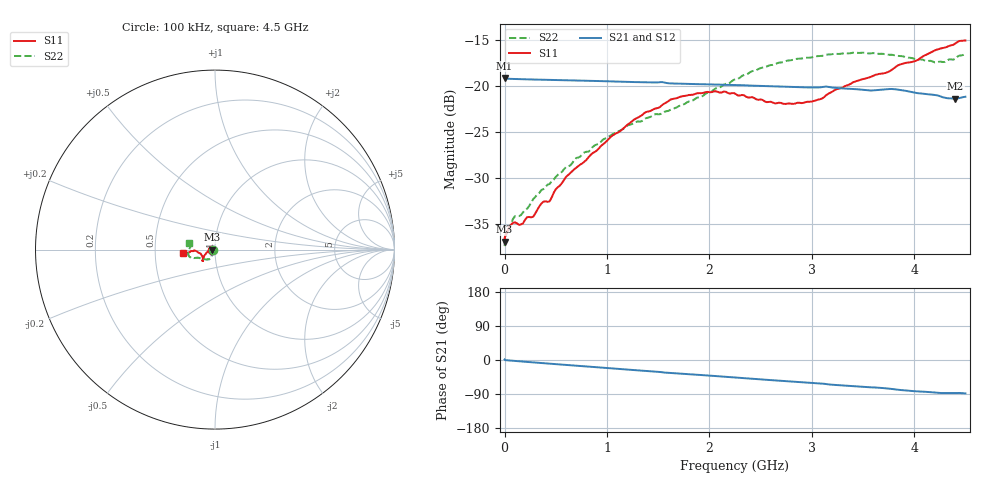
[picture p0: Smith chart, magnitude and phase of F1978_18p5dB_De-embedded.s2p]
! Integrated Device Technology
! Corporate Headquarters
! 6024 Silver Creek Valley Road
! San Jose, CA 95138  USA
! Phone:  1-408-284-8200
! Toll Free:  1-800-223-1366
! Webpage:  http://www.idt.com/
! Timing and RF Division
! 515 Groton Road, Suite 102
! Westford, MA 01886-6024
! Device:  F1978
! Description: 6-bit, 75 ohm, 0.5 dB Digital Step Attenuator
! Frequency:  5.0 MHz -  3.00 GHz
! Package:  4x4 mm QFN Plastic Package: 20 pin
! Ports:  2 RF, 11 DC
!  Pin  1  = D5 (16 dB)
!  Pin  2  = RF1  =  Port 1
!  Pin  3  = Serial Data In (DATA)
!  Pin  4  = Serial Clock (CLK)
!  Pin  5  = Serial Latch Enable (LE)
!  Pin  6  = VDD
!  Pin  7  = NC
!  Pin  8  = NC
!  Pin  9  = NC
!  Pin 10  = GND
!  Pin 11  = GND
!  Pin 12  = NC
!  Pin 13  = VMODE
!  Pin 14  = RF2  =  Port 2
!  Pin 15  = D4 (8 dB)
!  Pin 16  = D3 (4 dB)
!  Pin 17  = D2 (2 dB)
!  Pin 18  = NC
!  Pin 19  = D1 (1 dB)
!  Pin 20  = D0 (0.5 dB)
! State:  37
! Atten State:  18.5 dB
! Voltage:  +3.30 Volts
! Current:  0.565 mA
! Data:  The device was measured on a F1975 evaluation board which has
!  individual transmission lines to the RF pins.  Data was collected
!  using a calibrated network analyzer.  The evaluation board was
!  de-embedded using Automatic Fixture Removal (AFR).
!  The reference plane is the edge of the package pin.
! Misc:
!  Action Tracker AT0416
! Date Measured:  2018-02-08
! Date:  2018-03-26  MJV
! Note:
!  Integrated Device Technology supplies this data as a sample of measured
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# GHz S dB R 75
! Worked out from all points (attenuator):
!   291 points, 100 kHz to 4.5 GHz, reference 75 ohm
!   highest |S21| = -19.12 dB at 100 kHz (marker M1); lowest = -21.4 dB at 4.4 GHz (marker M2)
!   lowest |S11| = -36.9 dB at 100 kHz (marker M3), VSWR 1.03, Z = 72.9 - j0.00663 ohm
!   |S11| at or under -10 dB: start of sweep to end of sweep
!   |S22| runs from -37.4 to -16.4 dB; largest |S21 - S12| = 0.00018
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0.0001  -36.94 -179.8  -19.12 1.2  -19.12 1.2  -37.44 -178.3
0.003  -36.47 -178.4  -19.17 0.7  -19.15 0.7  -36.63 -177.0
0.013  -36.15 -178.0  -19.19 -0.5  -19.19 -0.5  -36.15 -173.0
0.1  -34.83 -174.8  -19.23 -2.4  -19.23 -2.4  -34.18 -155.7
0.16  -35.08 -176.1  -19.26 -3.8  -19.26 -3.7  -34.05 -146.1
0.22  -34.28 -177.8  -19.27 -5.1  -19.27 -5.0  -33.36 -139.0
0.28  -34.23 -178.8  -19.29 -6.3  -19.29 -6.3  -32.32 -135.7
0.36  -32.78 -178.5  -19.31 -8.0  -19.31 -8.0  -31.32 -128.0
0.44  -32.55 -177.6  -19.33 -9.6  -19.33 -9.6  -30.67 -122.8
0.6  -29.89 -173.9  -19.38 -13.0  -19.38 -13.0  -28.81 -119.5
0.76  -28.41 -166.9  -19.42 -16.3  -19.41 -16.3  -27.44 -118.2
1.26  -23.69 -151.9  -19.57 -26.5  -19.56 -26.5  -24.05 -121.0
1.52  -22.26 -143.7  -19.57 -31.7  -19.57 -31.7  -23.06 -128.4
1.62  -21.47 -142.3  -19.71 -34.1  -19.71 -34.0  -22.59 -131.9
1.88  -20.79 -138.5  -19.79 -38.9  -19.79 -38.9  -21.26 -143.4
2.26  -20.89 -138.2  -19.89 -46.3  -19.89 -46.3  -19.25 -154.9
2.64  -21.89 -147.8  -20.04 -53.8  -20.03 -53.8  -17.63 -159.1
3.02  -21.63 -164.1  -20.15 -60.9  -20.14 -60.9  -16.82 -162.7
3.76  -18.39 -176.1  -20.32 -75.7  -20.32 -75.7  -16.60 -176.5
4.2  -16.13 -173.3  -20.97 -85.7  -20.97 -85.7  -17.43 171.0
4.4  -15.38 -171.5  -21.38 -87.2  -21.38 -87.2  -17.03 167.8
4.5  -15.04 -173.3  -21.16 -88.2  -21.16 -88.2  -16.42 166.5
